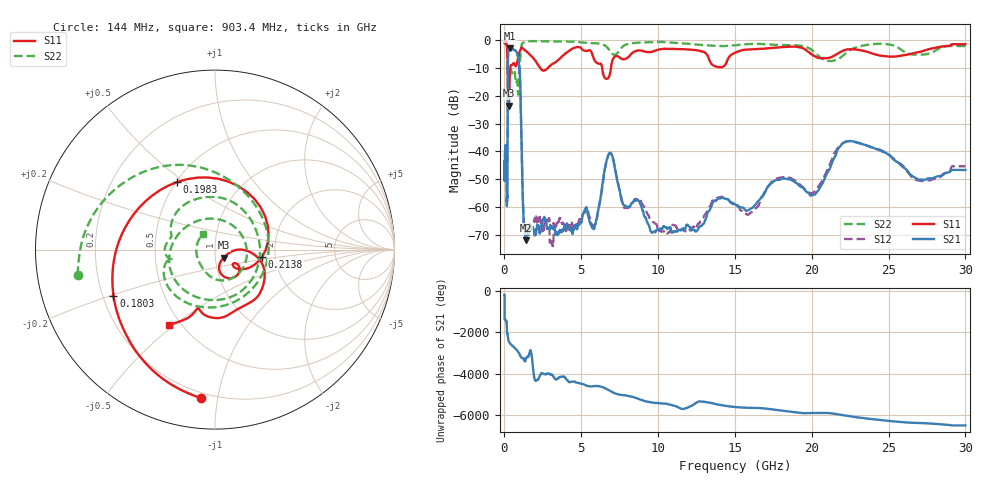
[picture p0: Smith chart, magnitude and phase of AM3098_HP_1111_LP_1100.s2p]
! Date/Time: Thu, Feb 28, 2019 8:48 AM
! Network Analyzer: Agilent Technologies E8364B Rev: A.07.50.67
! Sweep from 0.010 to 30.000 GHz, 1601 Points, Sweep Type: LOG
! Power Supply: 5.022 V, 0.001 A
# Hz S DB R 50
!freq MagS11 AngS11 MagS21 AngS21 MagS12 AngS12 MagS22 AngS22
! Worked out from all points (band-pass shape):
!   1601 points, 10 MHz to 30 GHz, reference 50 ohm
!   highest |S21| = -3.09 dB at 337.1 MHz (marker M1); lowest = -71.8 dB at 1.41 GHz (marker M2)
!   |S21| within 3 dB of the highest: 228.4 MHz to 888.2 MHz (659.8 MHz wide, 118 % of centre)
!   lowest |S11| = -23.6 dB at 293 MHz (marker M3), VSWR 1.14, Z = 54.9 - j4.98 ohm
!   |S11| at or under -10 dB: 210.1 MHz to 377.5 MHz (167.4 MHz wide, 57 % of centre); 2.323 GHz to 2.838 GHz (515.4 MHz wide, 20 % of centre); 6.358 GHz to 6.937 GHz (579.2 MHz wide, 8.71 % of centre)
!   |S22| runs from -19.6 to -0.5 dB; largest |S21 - S12| = 0.01
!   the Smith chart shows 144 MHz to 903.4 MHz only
!   S11 on the Smith chart (normalised r, x): 144 MHz: 0.17, -0.90; 180.3 MHz: 0.24, -0.20; 198.3 MHz: 0.51, +0.47; 213.8 MHz: 1.71, -0.14; 903.4 MHz: 0.43, -0.48
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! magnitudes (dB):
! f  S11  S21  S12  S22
! 10 MHz  -0.4  -45.3  -45.6  -0.6
! 38.04 MHz  -0.2  -41.3  -40.7  -0.7
! 144 MHz  -1.6  -53.8  -54.4  -2.2
! 144.7 MHz  -1.6  -53.9  -54.0  -2.2
! 180.3 MHz  -4.1  -55.9  -55.7  -5.4
! 198.3 MHz  -7.3  -36.8  -36.3  -10.4
! 213.8 MHz  -11.5  -12.8  -12.7  -9.4
! 293 MHz  -23.6  -3.3  -3.2  -11.8
! 337.1 MHz  -13.1  -3.1  -3.1  -11.2
! 550.5 MHz  -8.7  -3.4  -3.4  -11.4
! 903.4 MHz  -6.2  -6.6  -6.5  -19.2
! 1.024 GHz  -3.9  -15.3  -15.3  -6.9
! 1.251 GHz  -3.4  -65.2  -64.6  -0.9
! 1.41 GHz  -4.0  -71.8  -67.7  -0.6
! 2.084 GHz  -8.1  -67.6  -64.8  -0.5
! 5.783 GHz  -6.3  -67.8  -66.4  -1.2
! 6.855 GHz  -12.4  -40.6  -40.5  -3.9
! 7.926 GHz  -6.7  -59.7  -60.0  -1.7
! 11.77 GHz  -3.4  -67.9  -68.5  -1.3
! 20.1 GHz  -5.6  -55.5  -54.7  -4.0
! 22.56 GHz  -3.4  -36.3  -36.4  -3.5
! 30 GHz  -1.6  -46.6  -45.3  -2.2
